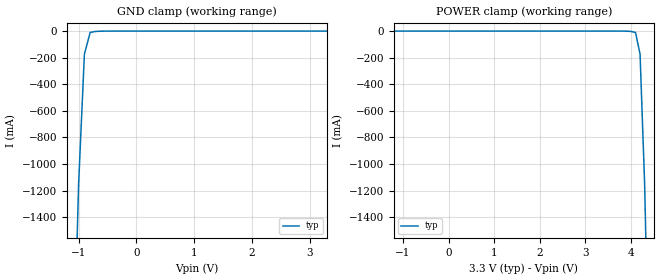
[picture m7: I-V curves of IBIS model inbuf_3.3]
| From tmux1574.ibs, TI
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| inbuf_3.3
[Model]   inbuf_3.3
Model_type   Input
Vinl = 0.45
Vinh = 1.2
|   typ   min   max
C_comp   2.533030e-12   NA   NA
[Voltage Range]   3.3   NA   NA
[Temperature Range]   27   NA   NA
[Power Clamp Reference]   3.3   NA   NA
[GND Clamp Reference]   0   NA   NA
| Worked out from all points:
|   GND clamp passes 1 mA (typ) near -0.62 V on its own axis
[GND Clamp]
|   Voltage   I(typ)   I(min)   I(max)
-6.6V     -112.6A    NA         NA
-1.1V     -2.712A    NA         NA
-1V       -1.15A     NA         NA
-900mV    -174.1mA   NA         NA
-800mV    -10.51mA   NA         NA
-700mV    -2.277mA   NA         NA
-500mV    -96.28uA   NA         NA
3.3V      550.1nA    NA         NA
[POWER Clamp]
|   Voltage   I(typ)   I(min)   I(max)
-3.3V     1.1uA      NA         NA
3.8V      -96.28uA   NA         NA
4V        -2.277mA   NA         NA
4.1V      -10.51mA   NA         NA
4.2V      -174.1mA   NA         NA
4.3V      -1.15A     NA         NA
4.4V      -2.712A    NA         NA
6.6V      -45.91A    NA         NA
